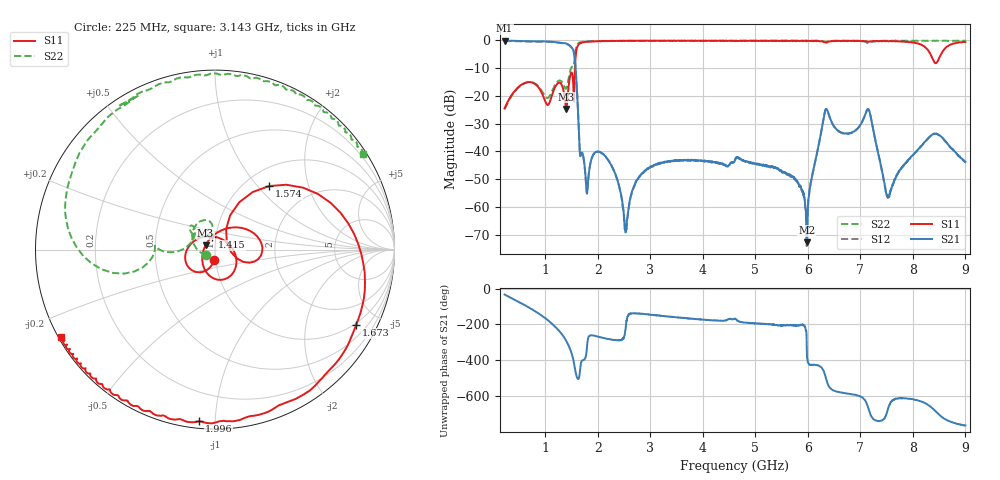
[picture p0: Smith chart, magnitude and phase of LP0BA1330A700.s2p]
!Agilent Technologies,E8358A,US41080443,A.07.50.56
!Agilent E8358A: A.07.50.56
!Date: Monday, March 28, 2016 13:01:08
!Correction: S11(Full 2 Port(1,2))
!S21(Full 2 Port(1,2))
!S12(Full 2 Port(1,2))
!S22(Full 2 Port(1,2))
!S2P File: Measurements: S11, S21, S12, S22:
# Hz S  dB  R 50
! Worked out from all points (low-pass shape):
!   1601 points, 225 MHz to 9 GHz, reference 50 ohm
!   highest |S21| = -0.05 dB at 225 MHz (marker M1); lowest = -72.7 dB at 5.978 GHz (marker M2)
!   |S21| within 3 dB of the highest: start of sweep to 1.521 GHz
!   lowest |S11| = -24.7 dB at 1.399 GHz (marker M3), VSWR 1.12, Z = 45 + j2.26 ohm
!   |S11| at or under -10 dB: start of sweep to 1.565 GHz
!   |S22| runs from -24.8 to 0.0 dB; largest |S21 - S12| = 0.014
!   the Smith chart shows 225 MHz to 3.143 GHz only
!   S11 on the Smith chart (normalised r, x): 225 MHz: 0.98, -0.12; 1.415 GHz: 0.96, +0.14; 1.574 GHz: 1.28, +1.15; 1.673 GHz: 0.92, -3.78; 1.996 GHz: 0.04, -0.91; 3.143 GHz: 0.01, -0.26
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2.25e8  -24.50 -95.4  -0.05 -33.5  -0.16 -33.4  -24.80 -150.8
6.582656e8  -15.06 -144.7  -0.31 -100.7  -0.42 -100.5  -15.13 124.5
1.031203e9  -23.11 82.8  -0.38 -172.3  -0.49 -172.1  -20.76 115.2
1.398656e9  -24.72 154.5  -1.12 68.6  -1.22 68.7  -17.31 159.5
1.415109e9  -22.66 103.9  -1.24 59.5  -1.34 59.6  -16.45 171.2
1.574156e9  -6.65 49.6  -9.12 -101.1  -9.24 -101.2  -3.90 -170.0
1.672875e9  -1.00 -28.1  -41.43 -63.1  -41.50 -62.9  -0.63 142.8
1.689328e9  -0.85 -34.1  -40.46 -44.9  -40.58 -45.8  -0.57 138.1
1.996453e9  -0.35 -95.3  -40.05 93.1  -40.07 92.8  -0.20 101.3
2.533922e9  -0.13 -130.5  -68.78 153.0  -68.95 151.7  -0.19 62.5
3.142688e9  -0.09 -150.4  -44.39 -149.6  -44.68 -149.1  -0.16 32.8
3.153656e9  -0.14 -150.6  -44.20 -150.3  -44.51 -150.7  -0.11 32.2
4.6125e9  -0.22 -178.5  -43.19 -168.2  -43.21 -167.0  -0.11 -15.6
5.978109e9  -0.28 152.3  -72.68 43.4  -74.13 55.9  -0.07 -38.6
6.076828e9  -0.15 149.6  -49.06 -66.0  -49.51 -64.2  -0.12 -39.4
6.345562e9  -0.77 145.3  -24.67 -141.1  -24.77 -140.3  -0.51 -42.3
7.140797e9  -0.50 132.0  -24.79 63.7  -24.79 63.8  -0.96 -53.8
7.541156e9  -0.32 125.6  -56.41 64.3  -56.64 62.9  -0.09 -56.9
8.144438e9  -1.40 92.4  -38.31 93.1  -38.44 93.0  -0.15 -66.1
8.369297e9  -6.36 19.9  -33.95 54.5  -33.98 55.0  -0.13 -68.8
8.533828e9  -5.09 -116.5  -34.57 9.7  -34.72 9.5  -0.16 -71.9
9e9  -0.50 168.9  -43.78 -41.8  -43.84 -42.0  -0.17 -78.5
